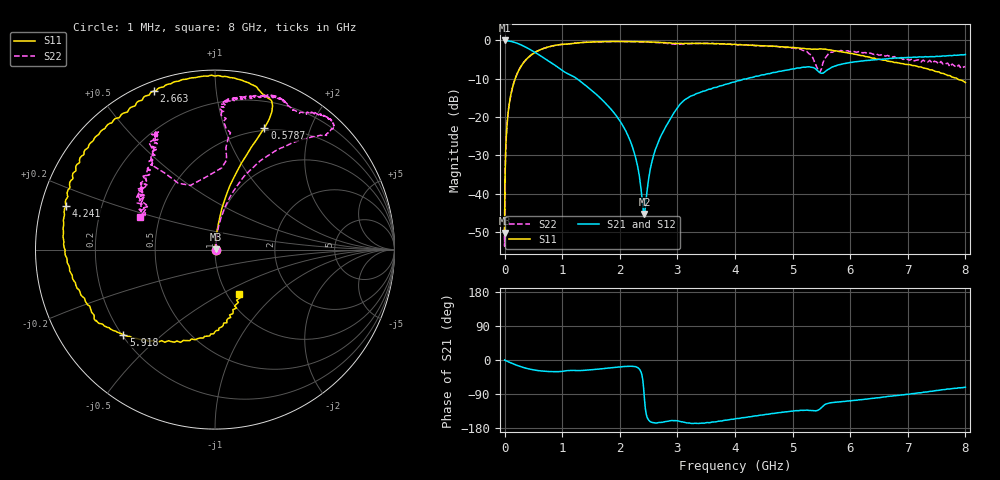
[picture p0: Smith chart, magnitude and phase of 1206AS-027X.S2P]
!s-Parameter Generated by FASTRON Sdn. Bhd.
!FASTRON P/N : 1206AS-027X
!Keysight Technologies: E5071C_MY46733604_B.14.02
!Date: Wed Nov 15 09:50:11 2023
!Version  :Rev00  Wed Nov 15 09:50:11 2023
!Data & Calibration Information:
!Freq  S11:SOLT2(ON)  S21:SOLT2(ON)  S12:SOLT2(ON)  S22:SOLT2(ON)
!PortZ  Port1:50+j0  Port2:50+j0
!When reading reference impedance value at option line is always used.
! Remarks : This data is being provided solely for informational purposes.
# Hz S dB R 50
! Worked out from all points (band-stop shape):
!   1601 points, 1 MHz to 8 GHz, reference 50 ohm
!   highest |S21| = -0.01 dB at 6.301 MHz (marker M1); lowest = -45.4 dB at 2.428 GHz (marker M2)
!   |S21| within 3 dB of the highest: start of sweep to 515.5 MHz
!   lowest |S11| = -50.3 dB at 1.541 MHz (marker M3), VSWR 1.01, Z = 50.3 + j0.0814 ohm
!   |S11| at or under -10 dB: start of sweep to 184.8 MHz; 7.859 GHz to end of sweep
!   |S22| runs from -53.8 to -0.3 dB; largest |S21 - S12| = 0.0066
!   S11 on the Smith chart (normalised r, x): 1 MHz: 1.01, -0.00; 578.7 MHz: 0.47, +1.38; 2.663 GHz: 0.04, +0.68; 4.241 GHz: 0.07, +0.14; 5.918 GHz: 0.21, -0.38; 8 GHz: 1.13, -0.61
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1000000  -47.34 -6.4  -0.03 -0.2  -0.04 -0.2  -49.08 -3.5
1541011  -50.31 15.4  -0.03 -0.3  -0.03 -0.2  -47.91 -2.0
4479405  -40.75 64.5  -0.04 -0.4  -0.04 -0.4  -41.17 68.7
6301378  -37.87 59.1  -0.01 -0.6  -0.03 -0.4  -41.23 68.7
2.00676e7  -28.49 81.6  -0.05 -1.5  -0.06 -1.5  -28.31 80.7
8.994653e7  -15.76 82.1  -0.18 -6.4  -0.19 -6.4  -15.81 79.9
4.006501e8  -4.60 70.8  -2.02 -22.8  -2.02 -22.8  -4.61 61.3
5.787206e8  -2.72 67.9  -3.58 -27.9  -3.59 -27.9  -2.71 54.2
1.024729e9  -1.00 69.8  -8.08 -29.5  -8.10 -29.5  -1.03 45.8
1.7949e9  -0.31 87.5  -17.06 -21.5  -17.08 -21.7  -0.31 47.3
2.125126e9  -0.31 96.2  -24.30 -17.0  -24.33 -17.2  -0.32 48.8
2.354847e9  -0.35 102.5  -37.03 -27.3  -37.04 -27.6  -0.35 51.2
2.428208e9  -0.38 104.7  -45.36 -102.0  -45.47 -102.0  -0.40 51.5
2.501569e9  -0.39 106.9  -36.13 -158.6  -36.14 -158.7  -0.44 52.9
2.662964e9  -0.48 111.2  -26.81 -165.5  -26.82 -165.7  -0.56 54.2
3.102129e9  -0.84 126.1  -15.85 -163.7  -15.87 -163.8  -0.91 63.3
4.240668e9  -1.26 163.7  -9.81 -150.0  -9.79 -150.1  -1.30 79.2
5.220382e9  -2.15 -160.1  -7.01 -132.6  -6.98 -132.8  -2.70 85.2
5.528293e9  -2.28 -149.1  -8.55 -121.4  -8.51 -121.7  -5.82 123.4
5.918038e9  -3.15 -137.1  -6.00 -109.1  -5.98 -109.4  -2.77 115.7
6.920464e9  -6.07 -97.4  -4.52 -92.0  -4.50 -92.6  -4.98 128.8
8e9  -11.00 -61.8  -3.69 -71.7  -3.67 -72.2  -6.82 156.9
